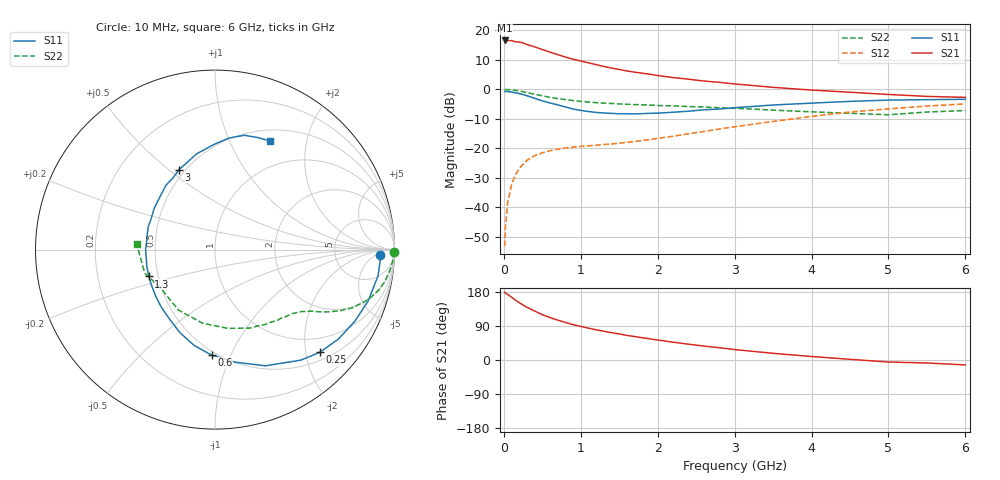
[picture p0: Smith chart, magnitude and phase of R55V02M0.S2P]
! SIEMENS Small Signal Semiconductors
! BFR183
! Si NPN RF Bipolar Junction Transistor in SOT23
! VCE = 5 V  IC = 2 mA
! Common Emitter S-Parameters:  May  1996
# GHz  S  MA  R  50
!  f  S11  S21  S12  S22
! GHz  MAG  ANG  MAG  ANG  MAG  ANG  MAG  ANG
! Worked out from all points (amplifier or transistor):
!   36 points, 10 MHz to 6 GHz, reference 50 ohm
!   highest |S21| = 16.6 dB at 10 MHz (marker M1)
!   |S21| within 3 dB of that: start of sweep to 490.3 MHz
!   unconditionally stable (mu >= 1): 1.395 GHz to 2.835 GHz
!   at 250 MHz: K = 0.23, MSG = 20.5 dB, |S12| = -25.3 dB
!   at 1.4 GHz: K = 1.00, MAG = 12.5 dB, |S12| = -18.5 dB
!   at 6 GHz: K = 0.90, MSG = 1.1 dB, |S12| = -4.9 dB
!   S11 on the Smith chart (normalised r, x): 10 MHz: 21, -8; 250 MHz: 0.66, -2.29; 600 MHz: 0.47, -0.85; 1.3 GHz: 0.44, -0.16; 3 GHz: 0.46, +0.54; 6 GHz: 0.64, +1.43
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0.01  0.9207 -1.8  6.744 178.9  0.0022 92.5  0.9955 -0.7
0.02  0.922 -3.9  6.652 177.0  0.0046 85.1  0.9898 -1.5
0.05  0.9203 -9.1  6.708 172.8  0.012 83.9  0.9922 -3.8
0.1  0.9 -18.6  6.704 165.8  0.0242 79.6  0.9783 -7.4
0.15  0.8754 -27.1  6.433 158.1  0.0355 74.9  0.9619 -10.8
0.2  0.8495 -35.9  6.338 151.4  0.0453 70.0  0.9393 -13.9
0.25  0.8177 -44.4  6.11 144.9  0.0544 65.7  0.9104 -16.8
0.3  0.7807 -52.0  5.757 139.2  0.0624 62.1  0.883 -19.2
0.4  0.7061 -66.5  5.251 129.3  0.0754 56.0  0.829 -23.1
0.5  0.6377 -79.7  4.726 119.5  0.0843 51.6  0.7758 -26.0
0.6  0.5878 -91.9  4.279 112.0  0.0913 48.1  0.7322 -28.2
0.8  0.503 -112.7  3.527 99.1  0.1015 43.8  0.6697 -31.1
0.9  0.4647 -122.6  3.248 93.4  0.1052 43.0  0.647 -32.1
1.1  0.421 -141.3  2.816 84.1  0.1106 43.0  0.6098 -34.4
1.3  0.3977 -157.9  2.447 75.9  0.1163 44.0  0.5848 -36.4
1.6  0.3867 179.8  2.048 64.9  0.1265 46.8  0.5587 -39.7
2.2  0.41 145.6  1.582 47.1  0.1603 52.9  0.5259 -48.6
3  0.4885 114.2  1.236 27.6  0.2326 54.3  0.4795 -65.7
3.5  0.5433 100.8  1.082 17.6  0.2859 51.0  0.445 -80.6
4.5  0.6262 82.9  0.894 1.8  0.4137 39.4  0.3934 -121.3
5.5  0.6686 68.8  0.76 -7.9  0.5214 25.0  0.413 -161.5
6  0.6783 63.2  0.732 -13.0  0.5672 15.7  0.4374 175.9
